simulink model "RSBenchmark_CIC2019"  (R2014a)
settings: Solver=ode23tb  SolverMode=SingleTasking  StartTime=0.0  StopTime=Tsim  FixedStep=0.1  MaxStep=20
PreLoadFcn:
  | addpath('Benchmark_files');
InitFcn:
  | Tm = 1;
StartFcn:
  | tic
StopFcn:
  | disp(['Simulation time lapse: ',num2str(toc),' s'])
undefined symbols (not defined in the file or in its folder): Av_Evap20_ini, Av_sat_max, Av_sat_min, Cond_inicial, h_c_in, h_c_out, I_Qe_good, I_TSH_good, mR, N_Main_ini, N_sat_max, N_sat_min, P_Qe_good, P_TSH_good, parameters, Parametros_de_simulacion, pc_in, pc_out, pe20, refr, secflux_c, tau, tau_evap
libraries: simulink x7

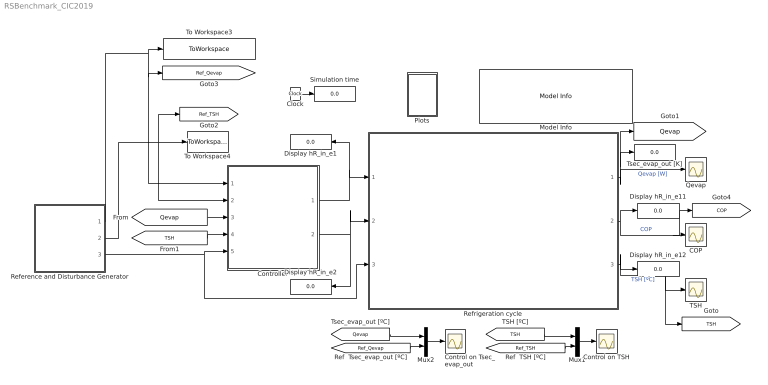
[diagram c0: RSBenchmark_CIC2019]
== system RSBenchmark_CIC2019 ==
  COP : Scope
  Clock : Clock
  Control on TSH : Scope
  Control on Tsec_evap_out : Scope
  Controller : Subsystem
  Display hR_in_e{1..2,11..12} (4 alike) : Display
  Model Info : simulink/Model-Wide Utilities/Model Info  InitialBlockCM=None  BlockCM=none  Frame=off  DisplayStringWithTags=|  HorizontalTextAlignment=Left  LeftAlignmentValue=0.02  SourceBlockDiagram=RSBenchmark_CIC2019  TagMaxNumber=20
      | Model Information:
      | Created: %<Created>
      | Modified Date: %<ModifiedDate>
      | Model Version: %<ModelVersion>
      | Model Name: %<ModelName>
      | Last ModificationDate: %<LastModificationDate>
  Mux1 : Mux  Inputs=2
  Mux2 : Mux  Inputs=2
  Plots : Subsystem
  Qevap : Scope
  Reference and Disturbance Generator : Subsystem
  Refrigeration cycle : Subsystem
  Simulation time : Display
  TSH : Scope
  To Workspace3 : ToWorkspace  VariableName=Ref_Qevap  SampleTime=Tm
  To Workspace4 : ToWorkspace  VariableName=Ref_TSH  SampleTime=Tm
  Tsec_evap_out [K] : Display
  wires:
  Refrigeration cycle/2(COP) -> [COP], COP/1, Display hR_in_e11/1  "COP"
  Refrigeration cycle/1(Qe) -> Tsec_evap_out [K]/1, [Qevap], Qevap/1  "Qevap [W]"
  Refrigeration cycle/3(TSH) -> [TSH], TSH/1, Display hR_in_e12/1  "TSH [ºC]"
  Clock/1 -> Simulation time/1
  Reference and Disturbance Generator/3(Disturbances) -> Controller/5(Disturbances), Refrigeration cycle/3(w)
  Reference and Disturbance Generator/1(Ref_Qevap) -> Controller/1(Ref Qevap), [Ref_Qevap], To Workspace3/1
  Controller/2(N) -> Refrigeration cycle/2(N), Display hR_in_e2/1
  Controller/1(Av) -> Refrigeration cycle/1(Av), Display hR_in_e1/1
  Reference and Disturbance Generator/2(Ref_TSH) -> Controller/2(Ref TSH), To Workspace4/1, [Ref_TSH]
  [Qevap] -> Controller/3(Qevap)
  [TSH] -> Controller/4(TSH)
  Mux1/1 -> Control on TSH/1
  Mux2/1 -> Control on Tsec_evap_out/1
  [Qevap] -> Mux2/1
  [TSH] -> Mux1/1
  [Ref_Qevap] -> Mux2/2
  [Ref_TSH] -> Mux1/2

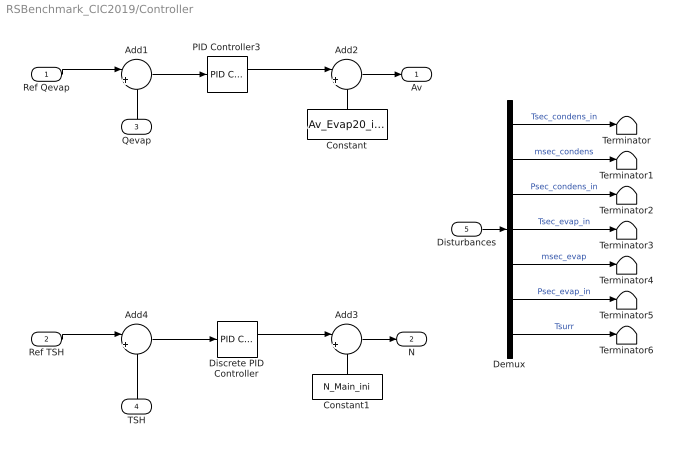
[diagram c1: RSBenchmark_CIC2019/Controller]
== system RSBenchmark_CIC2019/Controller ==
  Ref Qevap : Inport
  Ref TSH : Inport  Port=2
  Qevap : Inport  Port=3
  TSH : Inport  Port=4
  Disturbances : Inport  Port=5
  Add1 : Sum  Inputs=|+-
  Add2 : Sum  Inputs=|++
  Add3 : Sum  Inputs=|++
  Add4 : Sum  Inputs=|+-
  Constant : Constant  Value=Av_Evap20_ini
  Constant1 : Constant  Value=N_Main_ini
  Demux : Demux  Outputs=7
  Discrete PID Controller : simulink/Continuous/PID Controller  Controller=PI  TimeDomain=Continuous-time  SampleTime=-1  IntegratorMethod=Forward Euler  FilterMethod=Forward Euler  Form=Ideal  P=P_TSH_good  I=I_TSH_good  D=0  N=100  InitialConditionSource=internal  InitialConditionForIntegrator=0  InitialConditionForFilter=0  ExternalReset=none  LimitOutput=on  UpperSaturationLimit=N_sat_max - N_Main_ini  LowerSaturationLimit=N_sat_min - N_Main_ini  LinearizeAsGain=off  AntiWindupMode=back-calculation  Kb=1  TrackingMode=off  Kt=1  PParamMin=[]  PParamMax=[]  IParamMin=[]  IParamMax=[]  DParamMin=[]  DParamMax=[]  NParamMin=[]  NParamMax=[]  KbParamMin=[]  KbParamMax=[]  KtParamMin=[]  KtParamMax=[]  POutMin=[]  POutMax=[]  IOutMin=[]  IOutMax=[]  DOutMin=[]  DOutMax=[]  NOutMin=[]  NOutMax=[]  KbOutMin=[]  KbOutMax=[]  KtOutMin=[]  KtOutMax=[]  IntegratorOutMin=[]  IntegratorOutMax=[]  FilterOutMin=[]  FilterOutMax=[]  SumOutMin=[]  SumOutMax=[]  SumI1OutMin=[]  SumI1OutMax=[]  SumI2OutMin=[]  SumI2OutMax=[]  SumI3OutMin=[]  SumI3OutMax=[]  SumDOutMin=[]  SumDOutMax=[]  SaturationOutMin=[]  SaturationOutMax=[]  IntegratorContinuousStateAttributes=''  IntegratorStateMustResolveToSignalObject=off  IntegratorRTWStateStorageClass=Auto  FilterContinuousStateAttributes=''  FilterStateMustResolveToSignalObject=off  FilterRTWStateStorageClass=Auto
  PID Controller3 : simulink/Continuous/PID Controller  Controller=PI  TimeDomain=Continuous-time  SampleTime=-1  IntegratorMethod=Forward Euler  FilterMethod=Forward Euler  Form=Ideal  P=P_Qe_good  I=I_Qe_good  D=0  N=100  InitialConditionSource=internal  InitialConditionForIntegrator=0  InitialConditionForFilter=0  ExternalReset=none  LimitOutput=on  UpperSaturationLimit=100-Av_Evap20_ini  LowerSaturationLimit=Av_Evap20_ini-100  LinearizeAsGain=on  AntiWindupMode=none  Kb=1  TrackingMode=off  Kt=1  PParamMin=[]  PParamMax=[]  IParamMin=[]  IParamMax=[]  DParamMin=[]  DParamMax=[]  NParamMin=[]  NParamMax=[]  KbParamMin=[]  KbParamMax=[]  KtParamMin=[]  KtParamMax=[]  POutMin=[]  POutMax=[]  IOutMin=[]  IOutMax=[]  DOutMin=[]  DOutMax=[]  NOutMin=[]  NOutMax=[]  KbOutMin=[]  KbOutMax=[]  KtOutMin=[]  KtOutMax=[]  IntegratorOutMin=[]  IntegratorOutMax=[]  FilterOutMin=[]  FilterOutMax=[]  SumOutMin=[]  SumOutMax=[]  SumI1OutMin=[]  SumI1OutMax=[]  SumI2OutMin=[]  SumI2OutMax=[]  SumI3OutMin=[]  SumI3OutMax=[]  SumDOutMin=[]  SumDOutMax=[]  SaturationOutMin=[]  SaturationOutMax=[]  IntegratorContinuousStateAttributes=''  IntegratorStateMustResolveToSignalObject=off  IntegratorRTWStateStorageClass=Auto  FilterContinuousStateAttributes=''  FilterStateMustResolveToSignalObject=off  FilterRTWStateStorageClass=Auto
  Terminator{,1..6} (7 alike) : Terminator
  Av : Outport
  N : Outport  Port=2
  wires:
  TSH/1 -> Add4/2
  Qevap/1 -> Add1/2
  Add3/1 -> N/1
  Constant/1 -> Add2/2
  Constant1/1 -> Add3/2
  Ref TSH/1 -> Add4/1
  Ref Qevap/1 -> Add1/1
  Add2/1 -> Av/1
  Disturbances/1 -> Demux/1
  Demux/2 -> Terminator1/1  "msec_condens"
  Demux/3 -> Terminator2/1  "Psec_condens_in"
  Demux/4 -> Terminator3/1  "Tsec_evap_in"
  Demux/5 -> Terminator4/1  "msec_evap"
  Demux/6 -> Terminator5/1  "Psec_evap_in"
  Demux/7 -> Terminator6/1  "Tsurr"
  Demux/1 -> Terminator/1  "Tsec_condens_in"
  Add4/1 -> Discrete PID Controller/1
  Discrete PID Controller/1 -> Add3/1
  Add1/1 -> PID Controller3/1
  PID Controller3/1 -> Add2/1

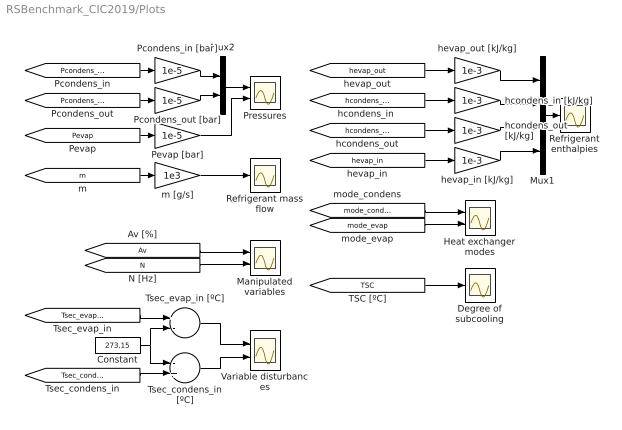
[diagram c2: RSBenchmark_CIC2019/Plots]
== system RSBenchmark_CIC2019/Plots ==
  Constant : Constant  Value=273.15
  Degree of subcooling : Scope
  Heat exchanger modes : Scope  NumInputPorts=2
  Manipulated variables : Scope  NumInputPorts=2
  Mux1 : Mux
  Mux2 : Mux  Inputs=2
  Pcondens_in [bar] : Gain  Gain=1e-5
  Pcondens_out [bar] : Gain  Gain=1e-5
  Pevap [bar] : Gain  Gain=1e-5
  Pressures : Scope  NumInputPorts=2
  Refrigerant enthalpies : Scope
  Refrigerant mass flow : Scope
  Tsec_condens_in [ºC] : Sum  Inputs=-+
  Tsec_evap_in [ºC] : Sum  Inputs=+-
  Variable disturbances : Scope  NumInputPorts=2
  hcondens_in [kJ/kg] : Gain  Gain=1e-3
  hcondens_out [kJ/kg] : Gain  Gain=1e-3
  hevap_in [kJ/kg] : Gain  Gain=1e-3
  hevap_out [kJ/kg] : Gain  Gain=1e-3
  m [g/s] : Gain  Gain=1e3
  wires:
  [m] -> m [g/s]/1
  Mux2/1 -> Pressures/1
  [Pcondens_in] -> Pcondens_in [bar]/1
  [Pevap] -> Pevap [bar]/1
  [hevap_in] -> hevap_in [kJ/kg]/1
  Mux1/1 -> Refrigerant enthalpies/1
  [hcondens_out] -> hcondens_out [kJ/kg]/1
  [hcondens_in] -> hcondens_in [kJ/kg]/1
  [hevap_out] -> hevap_out [kJ/kg]/1
  [mode_condens] -> Heat exchanger modes/1
  [mode_evap] -> Heat exchanger modes/2
  [Av] -> Manipulated variables/1
  [N] -> Manipulated variables/2
  [TSC] -> Degree of subcooling/1
  Pcondens_in [bar]/1 -> Mux2/1
  [Pcondens_out] -> Pcondens_out [bar]/1
  Pcondens_out [bar]/1 -> Mux2/2
  Pevap [bar]/1 -> Pressures/2
  m [g/s]/1 -> Refrigerant mass flow/1
  [Tsec_evap_in] -> Tsec_evap_in [ºC]/1
  Constant/1 -> Tsec_condens_in [ºC]/1, Tsec_evap_in [ºC]/2
  Tsec_evap_in [ºC]/1 -> Variable disturbances/1
  [Tsec_condens_in] -> Tsec_condens_in [ºC]/2
  Tsec_condens_in [ºC]/1 -> Variable disturbances/2
  hevap_out [kJ/kg]/1 -> Mux1/1
  hcondens_in [kJ/kg]/1 -> Mux1/2
  hcondens_out [kJ/kg]/1 -> Mux1/3
  hevap_in [kJ/kg]/1 -> Mux1/4

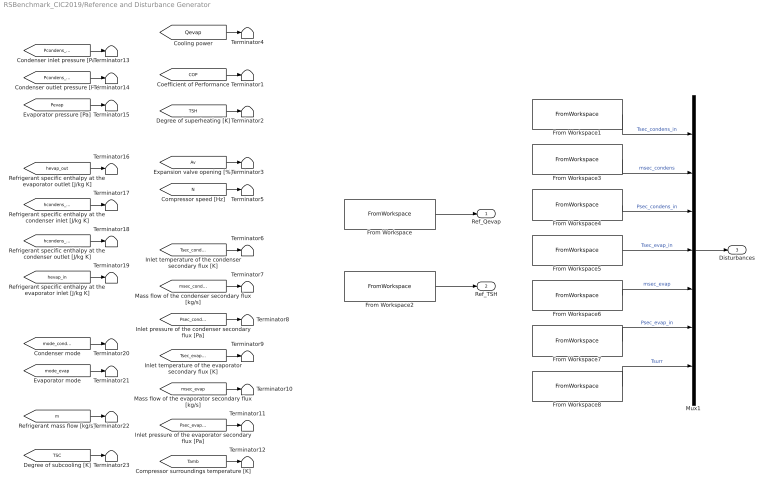
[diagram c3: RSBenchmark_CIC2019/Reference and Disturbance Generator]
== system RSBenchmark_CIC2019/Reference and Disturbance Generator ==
  From Workspace : FromWorkspace  VariableName=Ref_Qevap  SampleTime=Tm
  From Workspace1 : FromWorkspace  VariableName=Disturbances{1}  SampleTime=Tm
  From Workspace2 : FromWorkspace  VariableName=Ref_TSH  SampleTime=Tm
  From Workspace3 : FromWorkspace  VariableName=Disturbances{2}  SampleTime=Tm
  From Workspace4 : FromWorkspace  VariableName=Disturbances{3}  SampleTime=Tm
  From Workspace5 : FromWorkspace  VariableName=Disturbances{4}  SampleTime=Tm
  From Workspace6 : FromWorkspace  VariableName=Disturbances{5}  SampleTime=Tm
  From Workspace7 : FromWorkspace  VariableName=Disturbances{6}  SampleTime=Tm
  From Workspace8 : FromWorkspace  VariableName=Disturbances{7}  SampleTime=Tm
  Mux1 : Mux  Inputs=7
  Terminator{1..23} (23 alike) : Terminator
  Ref_Qevap : Outport
  Ref_TSH : Outport  Port=2
  Disturbances : Outport  Port=3
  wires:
  From Workspace1/1 -> Mux1/1  "Tsec_condens_in"
  From Workspace3/1 -> Mux1/2  "msec_condens"
  From Workspace4/1 -> Mux1/3  "Psec_condens_in"
  From Workspace5/1 -> Mux1/4  "Tsec_evap_in"
  From Workspace6/1 -> Mux1/5  "msec_evap"
  From Workspace7/1 -> Mux1/6  "Psec_evap_in"
  From Workspace8/1 -> Mux1/7  "Tsurr"
  From Workspace/1 -> Ref_Qevap/1
  From Workspace2/1 -> Ref_TSH/1
  Mux1/1 -> Disturbances/1
  [COP] -> Terminator1/1
  [TSH] -> Terminator2/1
  [Av] -> Terminator3/1
  [N] -> Terminator5/1
  [Tsec_condens_in] -> Terminator6/1
  [msec_condens] -> Terminator7/1
  [Psec_condens_in] -> Terminator8/1
  [Tsec_evap_in] -> Terminator9/1
  [msec_evap] -> Terminator10/1
  [Psec_evap_in] -> Terminator11/1
  [Tamb] -> Terminator12/1
  [Pcondens_in] -> Terminator13/1
  [Pcondens_out] -> Terminator14/1
  [Pevap] -> Terminator15/1
  [hevap_out] -> Terminator16/1
  [hcondens_in] -> Terminator17/1
  [hcondens_out] -> Terminator18/1
  [hevap_in] -> Terminator19/1
  [mode_condens] -> Terminator20/1
  [mode_evap] -> Terminator21/1
  [m] -> Terminator22/1
  [TSC] -> Terminator23/1
  [Qevap] -> Terminator4/1

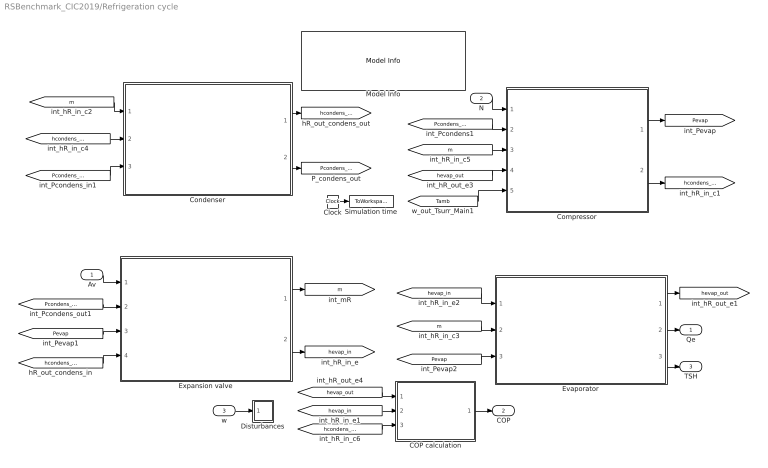
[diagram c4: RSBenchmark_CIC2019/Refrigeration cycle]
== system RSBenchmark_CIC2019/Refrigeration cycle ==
  Av : Inport
  N : Inport  Port=2
  w : Inport  Port=3
  COP calculation : Subsystem
  Clock : Clock
  Compressor : Subsystem
  Condenser : Subsystem
  Disturbances : Subsystem
  Evaporator : Subsystem
  Expansion valve : Subsystem
  Model Info : simulink/Model-Wide Utilities/Model Info  InitialBlockCM=None  BlockCM=none  Frame=off  DisplayStringWithTags=|  HorizontalTextAlignment=Left  LeftAlignmentValue=0.02  SourceBlockDiagram=RSBenchmark_CIC2019  TagMaxNumber=20
      | Model Information:
      | Created: %<Created>
      | Modified Date: %<ModifiedDate>
      | Model Version: %<ModelVersion>
      | Model Name: %<ModelName>
      | Last ModificationDate: %<LastModificationDate>
  Simulation time : ToWorkspace  VariableName=sim_t  SampleTime=Tm
  Qe : Outport
  COP : Outport  Port=2
  TSH : Outport  Port=3
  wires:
  [m] -> Evaporator/2(m1)
  [hcondens_in] -> Condenser/2(hcondens_in)
  [m] -> Compressor/3(m1)
  [m] -> Condenser/1(m)
  [Pevap] -> Evaporator/3(Pevap)
  [Pcondens_out] -> Expansion valve/2(P_in)
  [hcondens_out] -> Expansion valve/4(h_in)
  Expansion valve/2(h_out) -> [hevap_in]
  [Pcondens_out] -> Compressor/2(P_out)
  [Tamb] -> Compressor/5(Tamb)
  [Pcondens_in] -> Condenser/3(Pcondens_in)
  [hevap_in] -> Evaporator/1(hevap_in)
  Condenser/2(Pcondens_out) -> [Pcondens_out]
  Evaporator/1(hevap_out) -> [hevap_out]
  Expansion valve/1(m) -> [m]
  Condenser/1(hcondens_out) -> [hcondens_out]
  Compressor/2(h_out) -> [hcondens_in]
  [Pevap] -> Expansion valve/3(P_out)
  Compressor/1(P_in) -> [Pevap]
  [hevap_out] -> Compressor/4(h_in1)
  COP calculation/1(COP) -> COP/1
  [hevap_out] -> COP calculation/1(hevap_out)
  [hevap_in] -> COP calculation/2(hevap_in)
  [hcondens_in] -> COP calculation/3(hcondens_in)
  Av/1 -> Expansion valve/1(Av)
  Clock/1 -> Simulation time/1
  w/1 -> Disturbances/1(w)
  N/1 -> Compressor/1(N)
  Evaporator/2(Qe) -> Qe/1
  Evaporator/3(TSH) -> TSH/1

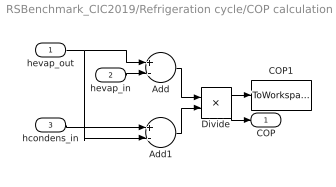
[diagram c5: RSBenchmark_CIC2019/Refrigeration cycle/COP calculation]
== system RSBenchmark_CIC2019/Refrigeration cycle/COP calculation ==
  hevap_out : Inport
  hevap_in : Inport  Port=2
  hcondens_in : Inport  Port=3
  Add : Sum  Inputs=+-
  Add1 : Sum  Inputs=+-
  COP1 : ToWorkspace  VariableName=COP  SampleTime=Tm
  Divide : Product  Inputs=*/
  COP : Outport
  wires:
  hevap_in/1 -> Add/2
  Add/1 -> Divide/1
  Add1/1 -> Divide/2
  hcondens_in/1 -> Add1/1
  hevap_out/1 -> Add1/2, Add/1
  Divide/1 -> COP1/1, COP/1

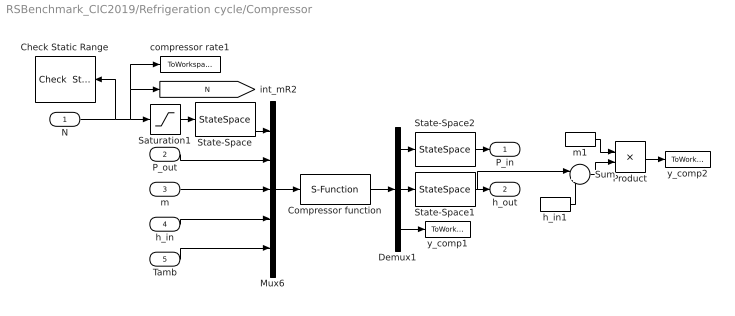
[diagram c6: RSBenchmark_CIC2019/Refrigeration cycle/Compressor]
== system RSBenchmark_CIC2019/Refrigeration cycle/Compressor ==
  N : Inport
  P_out : Inport  Port=2
  m : Inport  Port=3
  h_in : Inport  Port=4
  Tamb : Inport  Port=5
  Check Static Range : simulink/Model Verification/Check  Static Range  Description=N_sat_min <= u <= N_sat_max  max=N_sat_max  max_included=on  min=N_sat_min  min_included=on  enabled=on  callback=error(['Velocidad del compresor fuera de rango [30 , 50]'])  stopWhenAssertionFail=on  export=off  icon=graphic
  Compressor function : S-Function  FunctionName=Compressor  Parameters=parameters.comp,refr,pe20  EnableBusSupport=off
  Demux1 : Demux  Outputs=3
  Mux6 : Mux  Inputs=5
  Product : Product
  Saturation1 : Saturate  UpperLimit=N_sat_max  LowerLimit=N_sat_min
  State-Space : StateSpace  A=-1/tau_evap  B=1/tau_evap  D=0  X0=N_Main_ini
  State-Space1 : StateSpace  A=-1/tau  B=1/tau  D=0  X0=h_c_in
  State-Space2 : StateSpace  A=-1/tau  B=1/tau  D=0  X0=pe20
  Sum : Sum  Inputs=|+-
  compressor rate1 : ToWorkspace  VariableName=N  SampleTime=Tm
  h_in1 : InportShadow  Port=4
  m1 : InportShadow  Port=3
  y_comp1 : ToWorkspace  VariableName=Wcomp  SampleTime=Tm
  y_comp2 : ToWorkspace  VariableName=Qcomp  SampleTime=Tm
  P_in : Outport
  h_out : Outport  Port=2
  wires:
  Demux1/3 -> y_comp1/1
  Tamb/1 -> Mux6/5
  Mux6/1 -> Compressor function/1
  Compressor function/1 -> Demux1/1
  P_out/1 -> Mux6/2
  h_in/1 -> Mux6/4
  Demux1/2 -> State-Space1/1
  m/1 -> Mux6/3
  State-Space/1 -> Mux6/1
  State-Space1/1 -> h_out/1, Sum/1
  State-Space2/1 -> P_in/1
  Demux1/1 -> State-Space2/1
  m1/1 -> Product/1
  h_in1/1 -> Sum/2
  Sum/1 -> Product/2
  Product/1 -> y_comp2/1
  N/1 -> Check Static Range/1, compressor rate1/1, [N], Saturation1/1
  Saturation1/1 -> State-Space/1

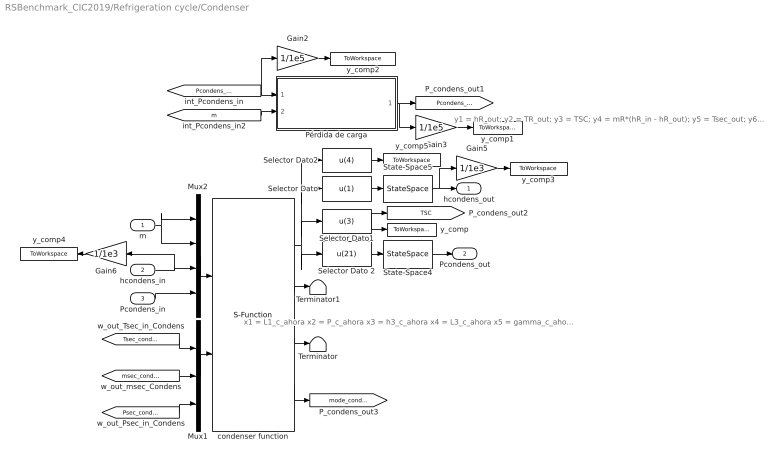
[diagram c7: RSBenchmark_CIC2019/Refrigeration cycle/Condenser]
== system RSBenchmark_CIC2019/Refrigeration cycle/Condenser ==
  note: x1 = L1_c_ahora x2 = P_c_ahora x3 = h3_c_ahora x4 = L3_c_ahora x5 = gamma_c_ahora
  note: y1 = hR_out; y2 = TR_out; y3 = TSC; y4 = mR*(hR_in - hR_out); y5 = Tsec_out; y6 = gammatot; y7 = Tsec_salida1; y8 = Tsec_salida2; y9 = Tsec_salida3; y10 = h1; y11 = h3til; y12 = L2; y13 = QR1; y14 = QR2; y15 = QR3; y16 = QR1_alt; y17 = QR2_alt; y18 = error; y19 = L1_c; y20 = gamma_c; y21 = Pc_out;
  m : Inport
  hcondens_in : Inport  Port=2
  Pcondens_in : Inport  Port=3
  Gain2 : Gain  Gain=1/1e5
  Gain3 : Gain  Gain=1/1e5
  Gain5 : Gain  Gain=1/1e3
  Gain6 : Gain  Gain=1/1e3
  Mux1 : Mux  Inputs=3
  Mux2 : Mux
  Pérdida de carga : Subsystem
  Selector Dato : Fcn  Expr=u(1)
  Selector Dato 2 : Fcn  Expr=u(21)
  Selector Dato1 : Fcn  Expr=u(3)
  Selector Dato2 : Fcn  Expr=u(4)
  State-Space4 : StateSpace  A=-1/tau  B=1/tau  D=0  X0=pc_out
  State-Space5 : StateSpace  A=-1/tau  B=1/tau  D=0  X0=h_c_out
  Terminator : Terminator
  Terminator1 : Terminator
  condenser function : S-Function  FunctionName=Condenser  Parameters=parameters.condens,refr,secflux_c,Cond_inicial,Parametros_de_simulacion  EnableBusSupport=off
  y_comp : ToWorkspace  VariableName=TSC  SampleTime=Tm
  y_comp1 : ToWorkspace  VariableName=Pcondens_in  SampleTime=Tm
  y_comp2 : ToWorkspace  VariableName=Pcondens_out  SampleTime=Tm
  y_comp3 : ToWorkspace  VariableName=hcondens_out  SampleTime=Tm
  y_comp4 : ToWorkspace  VariableName=hcondens_in  SampleTime=Tm
  y_comp5 : ToWorkspace  VariableName=Qcondens  SampleTime=Tm
  hcondens_out : Outport
  Pcondens_out : Outport  Port=2
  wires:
  Mux1/1 -> condenser function/2
  condenser function/3 -> Terminator/1
  condenser function/4 -> [mode_condens]
  condenser function/2 -> Terminator1/1
  condenser function/1 -> Selector Dato2/1, Selector Dato/1, Selector Dato1/1, Selector Dato 2/1
  [Psec_condens_in] -> Mux1/3
  [msec_condens] -> Mux1/2
  [Tsec_condens_in] -> Mux1/1
  Mux2/1 -> condenser function/1
  Selector Dato/1 -> State-Space5/1
  Selector Dato 2/1 -> State-Space4/1
  hcondens_in/1 -> Gain6/1, Mux2/3
  Pcondens_in/1 -> Mux2/4
  State-Space5/1 -> Gain5/1, hcondens_out/1
  State-Space4/1 -> Pcondens_out/1
  Pérdida de carga/1(Pcondens_in) -> Gain3/1, [Pcondens_in]
  Selector Dato1/1 -> y_comp/1, [TSC]
  [Pcondens_out] -> Gain2/1, Pérdida de carga/1(Pcondens_out)
  [m] -> Pérdida de carga/2(m)
  m/1 -> Mux2/2, Mux2/1
  Selector Dato2/1 -> y_comp5/1
  Gain2/1 -> y_comp2/1
  Gain3/1 -> y_comp1/1
  Gain5/1 -> y_comp3/1
  Gain6/1 -> y_comp4/1

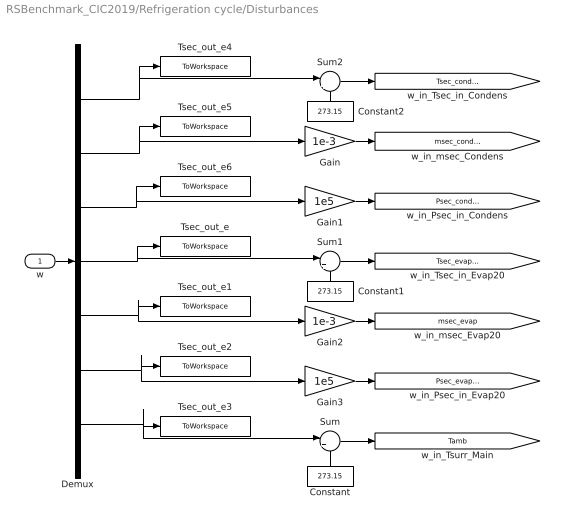
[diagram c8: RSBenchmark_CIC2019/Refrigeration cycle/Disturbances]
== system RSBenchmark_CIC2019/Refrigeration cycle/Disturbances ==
  w : Inport
  Constant : Constant  Value=273.15
  Constant1 : Constant  Value=273.15
  Constant2 : Constant  Value=273.15
  Demux : Demux  Outputs=7
  Gain : Gain  Gain=1e-3
  Gain1 : Gain  Gain=1e5
  Gain2 : Gain  Gain=1e-3
  Gain3 : Gain  Gain=1e5
  Sum : Sum  Inputs=|++
  Sum1 : Sum  Inputs=|++
  Sum2 : Sum  Inputs=|++
  Tsec_out_e : ToWorkspace  VariableName=Tsec_evap_in  SampleTime=Tm
  Tsec_out_e1 : ToWorkspace  VariableName=msec_evap  SampleTime=Tm
  Tsec_out_e2 : ToWorkspace  VariableName=Psec_evap  SampleTime=Tm
  Tsec_out_e3 : ToWorkspace  VariableName=Tsurr  SampleTime=Tm
  Tsec_out_e4 : ToWorkspace  VariableName=Tsec_condens_in  SampleTime=Tm
  Tsec_out_e5 : ToWorkspace  VariableName=msec_condens  SampleTime=Tm
  Tsec_out_e6 : ToWorkspace  VariableName=Psec_condens  SampleTime=Tm
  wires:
  w/1 -> Demux/1
  Constant/1 -> Sum/2
  Constant1/1 -> Sum1/2
  Constant2/1 -> Sum2/2
  Demux/1 -> Sum2/1, Tsec_out_e4/1
  Sum2/1 -> [Tsec_condens_in]
  Gain/1 -> [msec_condens]
  Demux/2 -> Gain/1, Tsec_out_e5/1
  Gain1/1 -> [Psec_condens_in]
  Demux/3 -> Gain1/1, Tsec_out_e6/1
  Demux/4 -> Tsec_out_e/1, Sum1/1
  Sum1/1 -> [Tsec_evap_in]
  Gain2/1 -> [msec_evap]
  Demux/5 -> Tsec_out_e1/1, Gain2/1
  Gain3/1 -> [Psec_evap_in]
  Demux/6 -> Tsec_out_e2/1, Gain3/1
  Sum/1 -> [Tamb]
  Demux/7 -> Tsec_out_e3/1, Sum/1

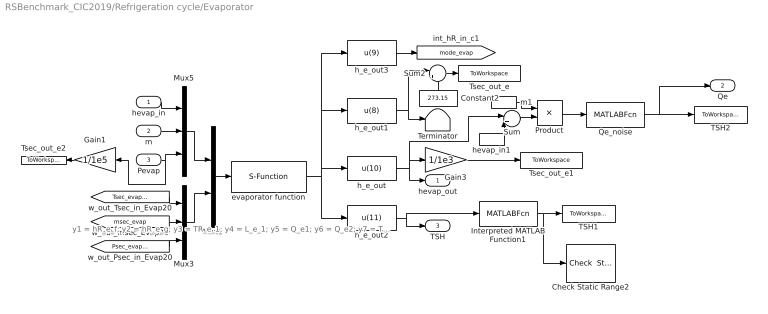
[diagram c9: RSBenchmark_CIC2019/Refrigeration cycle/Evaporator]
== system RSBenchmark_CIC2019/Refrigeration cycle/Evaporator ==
  note: y1 = hR_e_f; y2 = hR_e_g; y3 = TR_e_1; y4 = L_e_1; y5 = Q_e1; y6 = Q_e2; y7 = Tsec_out_e_1; y8 = Tsec_out_e; y9 = modo_e; y10 = hR_out_e; y11 = TSH
  hevap_in : Inport
  m : Inport  Port=2
  Pevap : Inport  Port=3
  Check Static Range2 : simulink/Model Verification/Check  Static Range  Description=TSH_sat_min <= u <= inf  max=inf  max_included=on  min=TSH_sat_min  min_included=on  enabled=on  callback=error(['Temperatura de sobrecalentamiento inferior a 0.5 ºC'])  stopWhenAssertionFail=on  export=off  icon=graphic
  Constant2 : Constant  Value=273.15
  Gain1 : Gain  Gain=1/1e5
  Gain3 : Gain  Gain=1/1e3
  Interpreted MATLAB Function1 : MATLABFcn  MATLABFcn=noise_TSH  OutputDimensions=1  OutputSignalType=real  SampleTime=0.5
  Mux1 : Mux  Inputs=2
  Mux3 : Mux  Inputs=3
  Mux5 : Mux  Inputs=3
  Product : Product
  Qe_noise : MATLABFcn  MATLABFcn=noise_Qe  OutputDimensions=1  OutputSignalType=real  Output1D=off  SampleTime=0.5
  Sum : Sum  Inputs=|+-
  Sum2 : Sum  Inputs=|+-
  TSH1 : ToWorkspace  VariableName=TSH  SampleTime=Tm
  TSH2 : ToWorkspace  VariableName=Qevap  SampleTime=Tm
  Terminator : Terminator
  Tsec_out_e : ToWorkspace  VariableName=Tsec_evap_out  SampleTime=Tm
  Tsec_out_e1 : ToWorkspace  VariableName=hevap_out  SampleTime=Tm
  Tsec_out_e2 : ToWorkspace  VariableName=Pevap  SampleTime=Tm
  evaporator function : S-Function  FunctionName=Evaporator  Parameters=parameters.evap, refr, secflux_evap20,hR_out_Evap20  EnableBusSupport=off
  h_e_out : Fcn  Expr=u(10)
  h_e_out1 : Fcn  Expr=u(8)
  h_e_out2 : Fcn  Expr=u(11)
  h_e_out3 : Fcn  Expr=u(9)
  hevap_in1 : InportShadow
  m1 : InportShadow  Port=2
  hevap_out : Outport
  Qe : Outport  Port=2
  TSH : Outport  Port=3
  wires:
  [Tsec_evap_in] -> Mux3/1
  [Psec_evap_in] -> Mux3/3
  [msec_evap] -> Mux3/2
  evaporator function/1 -> h_e_out3/1, h_e_out1/1, h_e_out/1, h_e_out2/1
  hevap_in/1 -> Mux5/1
  Mux1/1 -> evaporator function/1
  h_e_out1/1 -> Terminator/1, Sum2/1
  h_e_out2/1 -> Interpreted MATLAB Function1/1, TSH/1
  h_e_out/1 -> Sum/1, Gain3/1, hevap_out/1
  m/1 -> Mux5/2
  Pevap/1 -> Gain1/1, Mux5/3
  h_e_out3/1 -> [mode_evap]
  Mux5/1 -> Mux1/1
  Mux3/1 -> Mux1/2
  hevap_in1/1 -> Sum/2
  m1/1 -> Product/1
  Sum/1 -> Product/2
  Gain1/1 -> Tsec_out_e2/1
  Constant2/1 -> Sum2/2
  Sum2/1 -> Tsec_out_e/1
  Gain3/1 -> Tsec_out_e1/1
  Product/1 -> Qe_noise/1
  Qe_noise/1 -> TSH2/1, Qe/1
  Interpreted MATLAB Function1/1 -> Check Static Range2/1, TSH1/1

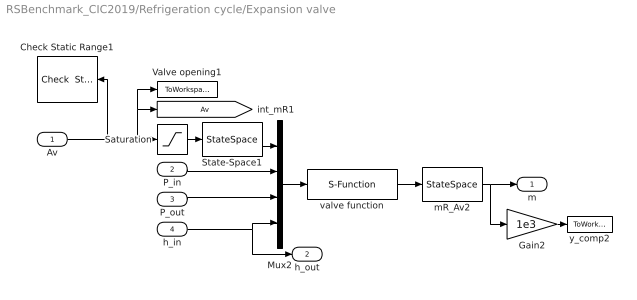
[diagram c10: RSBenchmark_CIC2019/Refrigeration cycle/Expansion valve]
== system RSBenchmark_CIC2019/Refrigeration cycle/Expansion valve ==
  Av : Inport
  P_in : Inport  Port=2
  P_out : Inport  Port=3
  h_in : Inport  Port=4
  Check Static Range1 : simulink/Model Verification/Check  Static Range  Description=Av_sat_min <= u <= Av_sat_max  max=Av_sat_max  max_included=on  min=Av_sat_min  min_included=on  enabled=on  callback=error(['Apertura de válvula fuera de rango [10,100]'])  stopWhenAssertionFail=on  export=off  icon=graphic
  Gain2 : Gain  Gain=1e3
  Mux2 : Mux
  Saturation : Saturate  UpperLimit=Av_sat_max  LowerLimit=Av_sat_min
  State-Space1 : StateSpace  A=-1/tau_evap  B=1/tau_evap  D=0  X0=Av_Evap20_ini
  Valve opening1 : ToWorkspace  VariableName=Av  SampleTime=Tm
  mR_Av2 : StateSpace  A=-1/tau  B=1/tau  D=0  X0=mR
  valve function : S-Function  FunctionName=Expansion_valve  Parameters=parameters.valv(1), 'R404a'  EnableBusSupport=off
  y_comp2 : ToWorkspace  VariableName=m  SampleTime=Tm
  m : Outport
  h_out : Outport  Port=2
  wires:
  Mux2/1 -> valve function/1
  Av/1 -> Check Static Range1/1, Valve opening1/1, [Av], Saturation/1
  valve function/1 -> mR_Av2/1
  P_out/1 -> Mux2/3
  P_in/1 -> Mux2/2
  h_in/1 -> h_out/1, Mux2/4
  mR_Av2/1 -> Gain2/1, m/1
  State-Space1/1 -> Mux2/1
  Saturation/1 -> State-Space1/1
  Gain2/1 -> y_comp2/1

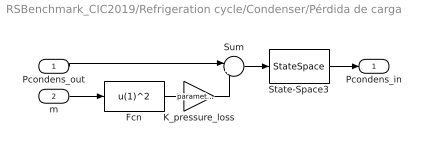
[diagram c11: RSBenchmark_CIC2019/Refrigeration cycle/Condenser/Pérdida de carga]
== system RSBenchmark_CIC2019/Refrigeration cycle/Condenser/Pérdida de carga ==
  Pcondens_out : Inport
  m : Inport  Port=2
  Fcn : Fcn  Expr=u(1)^2
  K_pressure_loss : Gain  Gain=parameters.condens.kperd
  State-Space3 : StateSpace  A=-1/tau  B=1/tau  D=0  X0=pc_in
  Sum : Sum  Inputs=|++
  Pcondens_in : Outport
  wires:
  K_pressure_loss/1 -> Sum/2
  Pcondens_out/1 -> Sum/1
  Sum/1 -> State-Space3/1
  State-Space3/1 -> Pcondens_in/1
  Fcn/1 -> K_pressure_loss/1
  m/1 -> Fcn/1
